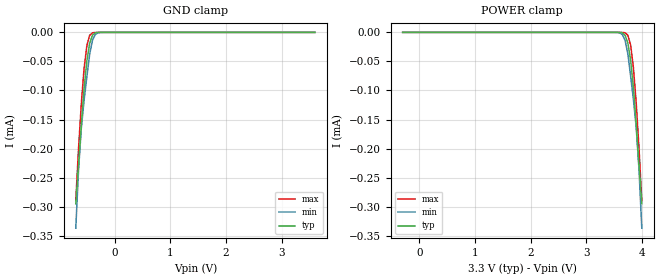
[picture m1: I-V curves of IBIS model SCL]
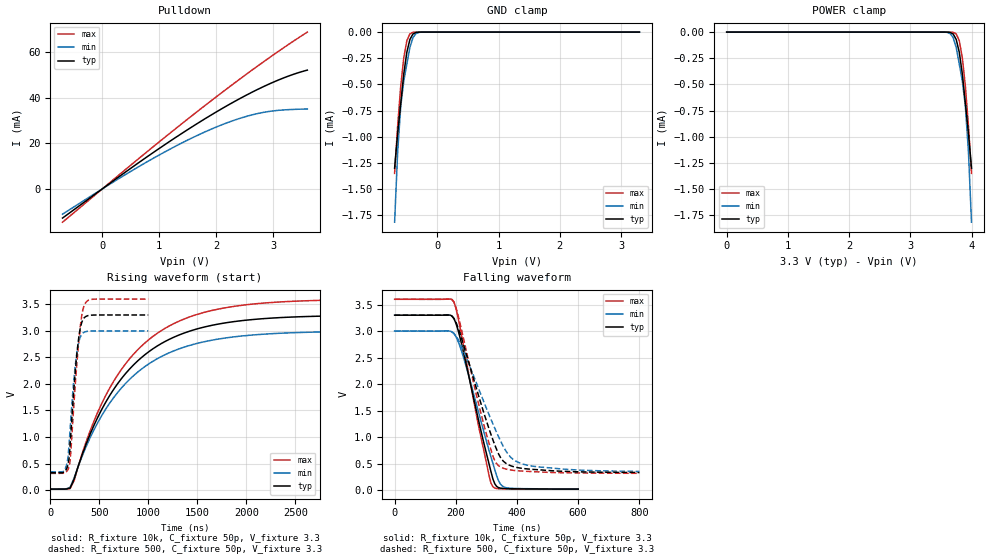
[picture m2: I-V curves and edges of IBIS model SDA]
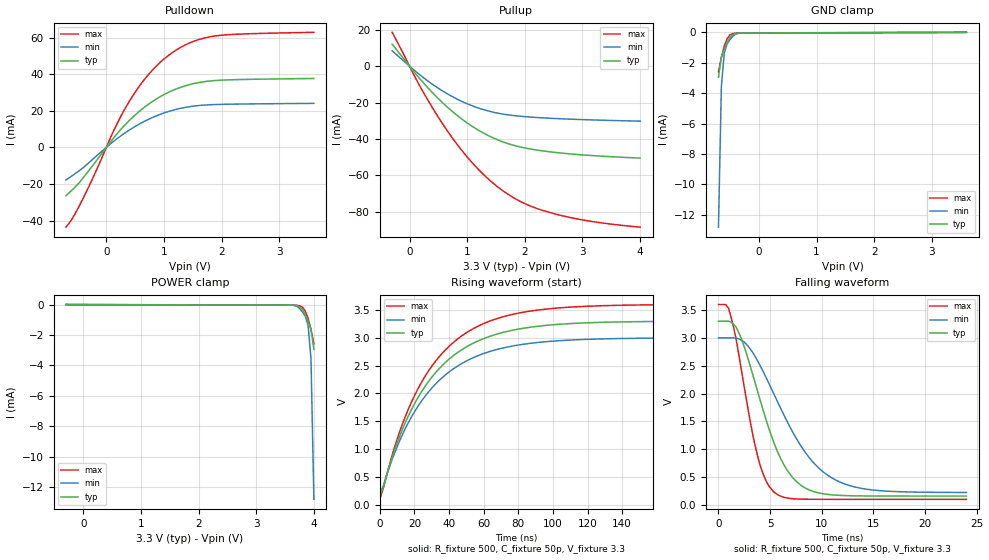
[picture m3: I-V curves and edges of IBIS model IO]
| PCA9538 - IBIS model
[IBIS Ver]   3.2
[Comment Char]   |_char
| VDD nom: 3.3v; min: 3v; max: 3.6v
[File name]   pca9538_3_3v.ibs
[File Rev]   1
[Date]   Aug 18, 2008 11:26:38 AM
[Source]
[Notes]
[Disclaimer]
(C) Copyright 2007 NXP Semiconductors
All rights reserved
NXP Semiconductors (NXP) does not warrant that this model and any other
accompanying information (Model) accurately or fully represents the
operating characteristics and specifications of the semiconductor
products to which the Model relates.  Moreover, the Model is furnished
on an "as is" and with "all faults" basis, and without support or
warranty of any kind.  NXP disclaims all warranties, whether expressed
or implied or statutory, including without limitation all implied
warranties of non-infringement, merchantability and fitness for any
purpose, and those arising from a course of dealing or usage of trade.
NXP does not convey any license under its or any third party's patents,
copyrights or other intellectual property or proprietary rights.
You and your company assume any and all risks and liability arising out
of the application or use of the Model.
In no event shall NXP be liable for any direct, indirect, special,
consequential or incidental damages, however caused, whether in
warranty, contract or tort (including negligence), strict liability or
other legal theory, including, without limitation, for lost profits,
business interruption, or corruption or loss of data or information,
arising out of or in connection with the use of or the inability to use
the Model, even if NXP has been advised of the possibility of such
damages.
NXP provides the Model as a courtesy to our customers. You and your
company shall not distribute, convey, sell, or give the Model to anyone
else without receiving prior written permission from NXP.
NXP reserves the right to make changes without notice to the Model to
improve reliability, function, or design.
Please be aware that your receipt and subsequent use of the Model shall
serve as acceptance of these terms and conditions.  If you do not
accept these terms, return or destroy the Model immediately.
[Copyright]
2008
| TSSOP16
[Component]   PCA9633PW
Si_location Pin
Timing_location Pin
[Manufacturer]   NXP Semiconductors
[Package]
R_pkg   3.92e-02   3.52e-02   4.56e-02
L_pkg   1.94n   1.65n   2.4n
C_pkg   0.446p   0.335p   0.771p
[Pin] signal_name   model_name   R_pin   L_pin   C_pin
1   A0   Addr   3.52E-02  2.40E-09  0.436E-12
2   A1   Addr   3.70E-02  1.93E-09  0.438E-12
3   RESETb   RESETb   4.56E-02  1.76E-09  0.345E-12
4   IO0   IO   4.00E-02  1.65E-09  0.335E-12
5   IO1   IO   4.00E-02  1.65E-09  0.335E-12
6   IO2   IO   4.56E-02  1.76E-09  0.345E-12
7   IO3   IO   3.70E-02  1.93E-09  0.438E-12
8   Vss   GND   3.52E-02  2.40E-09  0.452E-12
9   IO4   IO   3.52E-02  2.40E-09  0.452E-12
10   IO5   IO   3.70E-02  1.93E-09  0.438E-12
11   IO6   IO   4.56E-02  1.76E-09  0.345E-12
12   IO7   IO   4.00E-02  1.65E-09  0.771E-12
13   INTb   INT_OUT   4.00E-02  1.65E-09  0.771E-12
14   SCL   SCL   4.56E-02  1.76E-09  0.345E-12
15   SDA   SDA   3.70E-02  1.93E-09  0.438E-12
16   VDD   POWER   3.52E-02  2.40E-09  0.452E-12
| SO16
[Component]   PCA9633D16
Si_location Pin
Timing_location Pin
[Manufacturer]   NXP Semiconductors
[Package]
R_pkg   4.96e-02   3.94e-02   5.98e-02
L_pkg   2.52n   1.87n   3.16n
C_pkg   0.628p   0.494p   0.763p
[Pin] signal_name   model_name   R_pin   L_pin   C_pin
1   A0   Addr   5.98E-02  3.16E-09  7.63E-13
2   A1   Addr   4.55E-02  2.41E-09  6.04E-13
3   RESETb   RESETb   4.64E-02  1.93E-09  5.15E-13
4   IO0   IO   3.94E-02  1.87E-09  4.94E-13
5   IO1   IO   3.94E-02  1.87E-09  4.94E-13
6   IO2   IO   4.64E-02  1.93E-09  5.15E-13
7   IO3   IO   4.55E-02  2.41E-09  6.04E-13
8   Vss   GND   5.98E-02  3.16E-09  7.63E-13
9   IO4   IO   5.98E-02  3.16E-09  7.63E-13
10   IO5   IO   4.55E-02  2.41E-09  6.04E-13
11   IO6   IO   4.64E-02  1.93E-09  5.15E-13
12   IO7   IO   3.94E-02  1.87E-09  4.94E-13
13   INTb   INT_OUT   3.94E-02  1.87E-09  4.94E-13
14   SCL   SCL   4.64E-02  1.93E-09  5.15E-13
15   SDA   SDA   4.55E-02  2.41E-09  6.04E-13
16   VDD   POWER   5.98E-02  3.16E-09  7.63E-13
[Define Package Model]  HVQFN16
[Manufacturer]  ST-NXP Wireless
[OEM]  Unknown
[Description]  Full package model
|[Simulated] Chris Hunat
|[Approved] Wayne Nunn, Roger Real
[Number Of Pins]  16
[Pin Numbers]
|Pin Num   Terminal Name
1   | lead1:pin1
2   | lead2:pin2
3   | lead3:pin3
4   | lead4:pin4
5   | lead5:pin5
6   | lead6:pin6
7   | lead7:pin7
8   | lead8:pin8
9   | lead9:pin9
10   | lead10:pin10
11   | lead11:pin11
12   | lead12:pin12
13   | lead13:pin13
14   | lead14:pin14
15   | lead15:pin15
16   | lead16:pin16
[Model Data]
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[End Model Data]
[End Package Model]
| Models and submodels in the file (6): SCL (Input), SDA (I/O_open_drain), IO (I/O), RESETb (Input), INT_OUT (Open_drain), Addr (Input)
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[Model]   SCL
Model_type Input
Vinh=2.31
Vinl=0.99
C_comp   1.84p   1.81p   1.86p
[Temperature Range] 27   85   -40
[Voltage Range]   3.3   3   3.6
[GND Clamp]
-700mV    -295uA     -337uA     -289.5uA
-650mV    -228.6uA   -236.2uA   -199.5uA
-600mV    -158.8uA   -164.3uA   -122uA
-550mV    -96.13uA   -116.2uA   -61.46uA
-500mV    -48.62uA   -75.94uA   -22.35uA
-450mV    -18.67uA   -37.44uA   -5.001uA
-400mV    -4.926uA   -13.83uA   -710.6nA
-350mV    -920.5nA   -3.647uA   -77.67nA
-300mV    -138.4nA   -722.3nA   -7.551nA
-200mV    -2.42nA    -18.61nA   -62.47pA
3.6V      8.544pA    24.57pA    7.213pA
[POWER Clamp]
-300mV    8.544pA    24.57pA    7.213pA
3.5V      -2.42nA    -18.61nA   -62.47pA
3.6V      -138.4nA   -722.3nA   -7.551nA
3.65V     -920.5nA   -3.647uA   -77.68nA
3.7V      -4.926uA   -13.83uA   -710.6nA
3.75V     -18.67uA   -37.44uA   -5.001uA
3.8V      -48.62uA   -75.94uA   -22.35uA
3.85V     -96.13uA   -116.2uA   -61.46uA
3.9V      -158.8uA   -164.3uA   -122uA
3.95V     -228.6uA   -236.2uA   -199.5uA
4V        -295uA     -337uA     -289.5uA
[Model]   SDA
Model_type I/O_open_drain
Enable Active-High
Vinh=2.31
Vinl=0.99
Vref=3.3
Vmeas=1.65
Rref=10k
Cref=50p
C_comp   6.2p   6p   6.4p
[Temperature Range] 27   85   -40
[Voltage Range]   3.3   3   3.6
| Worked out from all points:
|   slope of the pulldown table from 0 to 0.495 V, typ, clamps not added: 55.4 ohm
|   GND clamp passes 1 mA (typ) near -0.65 V on its own axis
|   falling waveform, R_fixture 10k, C_fixture 50p, V_fixture 3.3: 20-80 % time 77.4ns typ, 85ns min, 72ns max; typ from 3.3 V to 0.019 V
|   falling waveform, R_fixture 500, C_fixture 50p, V_fixture 3.3: 20-80 % time 95.5ns typ, 114ns min, 82.3ns max; typ from 3.3 V to 0.332 V
|   rising waveform, R_fixture 10k, C_fixture 50p, V_fixture 3.3: 20-80 % time 704ns typ, 705ns min, 703ns max; typ from 0.018 V to 3.3 V
|   rising waveform, R_fixture 500, C_fixture 50p, V_fixture 3.3: 20-80 % time 74.8ns typ, 70.1ns min, 79.8ns max; typ from 0.327 V to 3.3 V
[Pulldown]
-700mV    -12.8mA    -11.11mA   -14.61mA
200mV     3.646mA    3.118mA    4.181mA
800mV     14.28mA    12.04mA    16.55mA
1.4V      24.35mA    20.14mA    28.62mA
1.9V      32.18mA    26.01mA    38.38mA
2.35V     38.65mA    30.34mA    46.89mA
2.75V     43.82mA    33.1mA     54.2mA
3.2V      48.75mA    34.59mA    62.06mA
3.6V      52mA       34.98mA    68.66mA
[GND Clamp]
-700mV    -1.302mA   -1.818mA   -1.351mA
-650mV    -970uA     -1.147mA   -895.5uA
-600mV    -683.7uA   -711.2uA   -519.4uA
-550mV    -399.4uA   -467.3uA   -244.7uA
-500mV    -192.3uA   -305.3uA   -82.59uA
-450mV    -70.46uA   -146.9uA   -17.18uA
-400mV    -17.84uA   -52.38uA   -2.302uA
-350mV    -3.222uA   -13.43uA   -238.8nA
-300mV    -468.9nA   -2.601uA   -22.09nA
-200mV    -7.684nA   -64.03nA   -166.2pA
3.3V      16.1pA     60.18pA    13.22pA
[POWER Clamp]
0V        16.1pA     60.18pA    13.22pA
3.5V      -7.684nA   -64.03nA   -166.2pA
3.6V      -468.9nA   -2.601uA   -22.09nA
3.65V     -3.222uA   -13.43uA   -238.8nA
3.7V      -17.84uA   -52.38uA   -2.302uA
3.75V     -70.46uA   -146.9uA   -17.18uA
3.8V      -192.3uA   -305.3uA   -82.59uA
3.85V     -399.4uA   -467.3uA   -244.7uA
3.9V      -683.7uA   -711.2uA   -519.4uA
3.95V     -970uA     -1.147mA   -895.5uA
4V        -1.302mA   -1.818mA   -1.351mA
[Falling Waveform]
R_fixture=10k
C_fixture=50p
V_fixture=3.3
V_fixture_min=3
V_fixture_max=3.6
0s        3.3V       3V         3.6V
193.9ns   3.235V     2.951V     3.546V
206.1ns   3.044V     2.825V     3.292V
224.2ns   2.622V     2.523V     2.751V
278.8ns   1.204V     1.373V     1.09V
309.1ns   482.8mV    739.1mV    262.9mV
321.2ns   210.3mV    502.9mV    63.21mV
339.4ns   48.05mV    179.7mV    26.56mV
363.6ns   28.33mV    46.21mV    22.3mV
600ns     18.89mV    20.72mV    17.62mV
[Falling Waveform]
R_fixture=500
C_fixture=50p
V_fixture=3.3
V_fixture_min=3
V_fixture_max=3.6
0s        3.3V       3V         3.6V
177.8ns   3.302V     3.001V     3.603V
193.9ns   3.24V      2.957V     3.547V
226.3ns   2.722V     2.612V     2.832V
299ns     1.324V     1.558V     1.077V
323.2ns   915mV      1.221V     607.3mV
339.4ns   685.5mV    1.011V     462.1mV
379.8ns   458.3mV    616.6mV    379.2mV
428.3ns   402.5mV    476.8mV    354.9mV
800ns     331.8mV    352.4mV    316.9mV
[Rising Waveform]
R_fixture=10k
C_fixture=50p
V_fixture=3.3
V_fixture_min=3
V_fixture_max=3.6
0s        17.92mV    18.99mV    17.1mV
202ns     37.47mV    51.51mV    26.79mV
242.4ns   202.9mV    225mV      173.8mV
444.4ns   1.215V     1.131V     1.295V
646.5ns   1.897V     1.742V     2.05V
929.3ns   2.496V     2.279V     2.712V
1.253us   2.874V     2.618V     3.13V
1.616us   3.092V     2.813V     3.371V
2.101us   3.22V      2.928V     3.512V
4us       3.297V     2.998V     3.597V
[Rising Waveform]
R_fixture=500
C_fixture=50p
V_fixture=3.3
V_fixture_min=3
V_fixture_max=3.6
0s        327.4mV    343.4mV    314.8mV
141.4ns   341.2mV    369.6mV    320.3mV
171.7ns   423.2mV    510.5mV    362.2mV
191.9ns   600.2mV    861.9mV    440.2mV
202ns     842.2mV    1.138V     542.1mV
232.3ns   1.69V      1.902V     1.377V
272.7ns   2.588V     2.611V     2.419V
313.1ns   3.11V      2.911V     3.187V
353.5ns   3.26V      2.981V     3.511V
1us       3.3V       3V         3.6V
[Ramp]
R_load=500
dV/dt_r   1.784E+0/6.455E-8   1.753E+0/6.240E-8   1.807E+0/6.654E-8
dV/dt_f   1.781E+0/9.604E-8   1.747E+0/1.237E-7   1.806E+0/7.725E-8
|[End   SDA
[Model]   IO
Model_type I/O
Enable Active-High
Polarity Non-Inverting
Vinh=2.31
Vinl=0.99
Vref=3.3
Vmeas=1.65
Rref=500
Cref=50p
C_comp   8p   7.8p   8.2p
[Temperature Range] 27   85   -40
[Voltage Range]   3.3   3   3.6
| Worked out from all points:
|   slope of the pulldown table from 0 to 0.495 V, typ, clamps not added: 28.2 ohm
|   slope of the pullup table from 0 to 0.495 V, typ, clamps not added: 28 ohm
|   GND clamp passes 1 mA (typ) near -0.59 V on its own axis
|   falling waveform, R_fixture 500, C_fixture 50p, V_fixture 3.3: 20-80 % time 3.36ns typ, 4.91ns min, 2.12ns max; typ from 3.3 V to 0.157 V
|   rising waveform, R_fixture 500, C_fixture 50p, V_fixture 3.3: 20-80 % time 35.7ns typ, 35.8ns min, 35.6ns max; typ from 0.157 V to 3.3 V
[Pullup]
-300mV    12.02mA    8.411mA    18.59mA
200mV     -7.686mA   -5.294mA   -12.12mA
600mV     -20.87mA   -14.14mA   -32.92mA
800mV     -26.39mA   -17.69mA   -41.9mA
1.05V     -32.28mA   -21.32mA   -51.72mA
1.25V     -36.19mA   -23.58mA   -58.48mA
1.5V      -40.1mA    -25.63mA   -65.58mA
1.9V      -44.25mA   -27.46mA   -73.96mA
2.15V     -45.8mA    -28.09mA   -77.51mA
2.4V      -46.93mA   -28.57mA   -80.11mA
3.1V      -48.98mA   -29.47mA   -85.02mA
4V        -50.51mA   -30.21mA   -88.46mA
[Pulldown]
-700mV    -26.42mA   -17.77mA   -43.6mA
-550mV    -22.05mA   -14.57mA   -36.77mA
-400mV    -16.62mA   -11.06mA   -27.75mA
150mV     6.068mA    3.88mA     10.55mA
350mV     13.13mA    8.458mA    22.56mA
500mV     17.69mA    11.45mA    30.15mA
700mV     22.87mA    14.86mA    38.63mA
1.05V     29.66mA    19.33mA    49.58mA
1.45V     34.38mA    22.29mA    57.17mA
1.85V     36.45mA    23.38mA    60.73mA
2.35V     37.11mA    23.71mA    61.98mA
3.6V      37.67mA    24.07mA    62.9mA
[GND Clamp]
-700mV    -2.949mA   -12.82mA   -2.591mA
-650mV    -1.618mA   -3.556mA   -1.65mA
-600mV    -1.097mA   -1.385mA   -902.1uA
-550mV    -647.3uA   -748.9uA   -419uA
-500mV    -317.7uA   -474.1uA   -166.2uA
-450mV    -139.5uA   -244.4uA   -69.6uA
-400mV    -64.91uA   -109.4uA   -44.89uA
-350mV    -42.27uA   -54.37uA   -40.06uA
-250mV    -35.59uA   -33.25uA   -38.46uA
3.6V      2.994uA    5.987uA    -359.9pA
[POWER Clamp]
-300mV    2.994uA    5.987uA    -359.9pA
3.55V     -35.59uA   -33.25uA   -38.46uA
3.65V     -42.27uA   -54.37uA   -40.06uA
3.7V      -64.91uA   -109.4uA   -44.89uA
3.75V     -139.5uA   -244.4uA   -69.59uA
3.8V      -317.7uA   -474.1uA   -166.2uA
3.85V     -647.3uA   -748.9uA   -419uA
3.9V      -1.097mA   -1.385mA   -902.1uA
3.95V     -1.618mA   -3.556mA   -1.65mA
4V        -2.949mA   -12.82mA   -2.591mA
[Falling Waveform]
R_fixture=500
C_fixture=50p
V_fixture=3.3
V_fixture_min=3
V_fixture_max=3.6
0s        3.3V       3V         3.6V
969.7ps   3.299V     3V         3.533V
2.182ns   3.004V     2.962V     2.462V
3.879ns   1.98V      2.556V     810.5mV
5.333ns   1.134V     2.003V     235.3mV
6.545ns   651.1mV    1.535V     126mV
7.758ns   384.8mV    1.124V     103mV
11.39ns   172.6mV    440.1mV    97.88mV
15.27ns   157.5mV    259.3mV    97.85mV
24ns      156.6mV    221.8mV    97.85mV
[Rising Waveform]
R_fixture=500
C_fixture=50p
V_fixture=3.3
V_fixture_min=3
V_fixture_max=3.6
0s        156.6mV    221.1mV    97.84mV
2.02ns    315.1mV    336.7mV    295.3mV
6.061ns   747.5mV    721.2mV    776mV
12.12ns   1.282V     1.197V     1.37V
22.22ns   1.935V     1.779V     2.095V
36.36ns   2.512V     2.293V     2.732V
52.53ns   2.88V      2.622V     3.139V
70.71ns   3.093V     2.814V     3.374V
96.97ns   3.226V     2.933V     3.519V
200ns     3.299V     2.999V     3.599V
[Ramp]
R_load=500
dV/dt_r   9.344E-3/1.616E-9   8.230E-3/1.816E-9   1.044E-2/1.370E-9
dV/dt_f   1.886E+0/4.373E-10   1.667E+0/7.399E-10   2.101E+0/2.343E-10
|[End   IO
